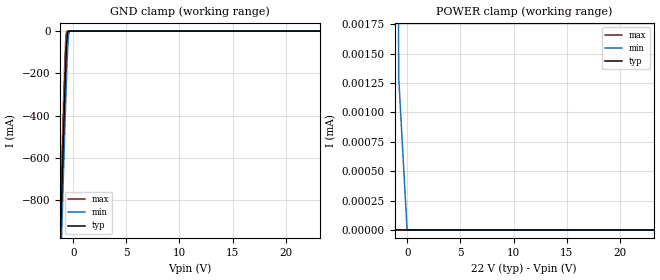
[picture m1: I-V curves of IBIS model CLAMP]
| Texas Instruments Incorporated
| TVS2200 22-V FlatClamp Surge Protection Device
[IBIS Ver]   4.1
[File name]   tvs2200.ibs
[File Rev]   1.0
[Date]   12/15/2017
[Source]
| Texas Instruments Incorporated.
| Analog-eLab Design Center, HPA
| 12500 TI Blvd
| Dallas, TX -75243
[Notes]   Revision History:
| Rev 1.0: 12/15/2017
| - Initial version of the model
| - Model generated from simulations in SPECTRE
| - Model matched to SPICE simulation
| - C_comp although listed in numerical order of value are
|   obtained from varying PVT conditions. For PVT conditions for
|   each specific value refer the buffer description under
|   respective [Model]. IBIS model user is responsible for using
|   appropriate C_comp to simulate for Signal Integrity.
[Disclaimer]
| This model is designed as an aid for customers of Texas Instruments.
| TI and its licensors and suppliers make no warranties, either expressed
| or implied, with respect to this  model, including the warranties of
| merchantability or fitness for a particular purpose. The model is
| provided solely on an "as is" basis. The entire risk as to its quality
| and performance is with the customer.
[Copyright]
(C) Copyright 2017 Texas Instruments Incorporated.All rights reserved.
|   TVS2200
[Component]   TVS2200DRV
[Manufacturer]   TI
[Package]   |6-pin SON DRV package
|   typ   min   max
R_pkg   0.03312   0.03141   0.03462
L_pkg   0.49614nH   0.44882nH   0.53669nH
C_pkg   0.15951pF   0.15201pF   0.17090pF
[Pin]  signal_name model_name   R_pin   L_pin  C_pin
1   GND   GND   NA   NA   NA
2   GND   GND   NA   NA   NA
3   GND   GND   NA   NA   NA
4   IN   CLAMP   NA   NA   NA
5   IN   CLAMP   NA   NA   NA
6   IN   CLAMP   NA   NA   NA
| Models and submodels in the file (1): CLAMP (Terminator)
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|   Model CLAMP
[Model]   CLAMP
Model_type   Terminator
|   typ   min   max
C_comp   7.937E-11   7.614E-11   7.937E-11
|Where Nom  PVT is Nominal Process, 22V,   40C
|   Fast PVT is Strong Process,  22.001V, -40C
|   Slow PVT is Weak Process,   21.999V, 125C
[Voltage Range]   22   21.999   22.001
[Temperature Range]   40   125   -40
[Power Clamp Reference]   22   21.999   22.001
[GND Clamp Reference]   0   0   0
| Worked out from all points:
|   GND clamp passes 1 mA (typ) near -0.46 V on its own axis
|   POWER clamp passes 1 mA (typ) near -4.58 V on its own axis
[GND Clamp]
|   Voltage   I(typ)   I(min)   I(max)
-22V      -41.05A    -41.05A    -41.08A
-1.342V   -1.233A    -1.405A    -1.08A
-1.144V   -887.3mA   -1.061A    -732.6mA
-1.078V   -773.4mA   -947.3mA   -618.3mA
-880mV    -439.9mA   -612.9mA   -285.5mA
-748mV    -231.3mA   -399.1mA   -88.66mA
-682mV    -137.1mA   -300.4mA   -21.83mA
-616mV    -58.95mA   -201.7mA   -2.174mA
-550mV    -13.29mA   -116.4mA   -289.7uA
-418mV    -135.2uA   -13.53mA   -14.53uA
-220mV    0A         -37.03uA   0A
44V       0A         0A         0A
[POWER Clamp]
|   Voltage   I(typ)   I(min)   I(max)
-22V      33.46A     36.29A     32.25A
-4.51V    259.3uA    2.975A     3.501uA
-4.444V   212uA      2.853A     1.457uA
-4.18V    98.63uA    2.365A     0A
-3.256V   2.454uA    702.8mA    0A
-3.19V    1.07uA     590mA      0A
-3.058V   0A         371.1mA    0A
-1.738V   0A         47.8uA     0A
-814mV    0A         1.301uA    0A
-22mV     0A         0A         0A
44V       0A         0A         0A
